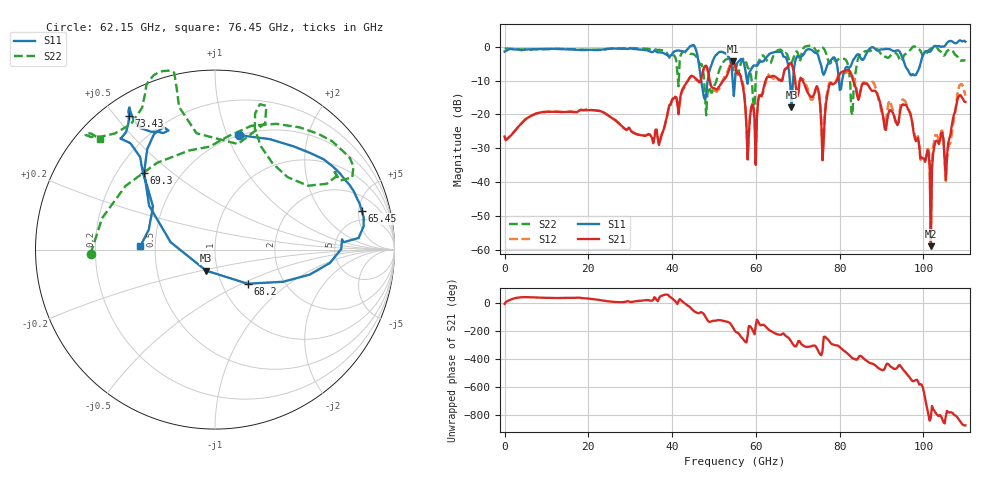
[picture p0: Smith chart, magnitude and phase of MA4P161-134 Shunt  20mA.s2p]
!Keysight Technologies,N5247B,US61255204,A.15.70.20
!Date: Friday, October 21, 2022 14:14:39
!Correction: S11(C  4-Port  )
!S31(C  4-Port  )
!S13(C  4-Port  )
!S33(C  4-Port  )
!S2P File: Measurements: S11, S31, S13, S33:
# Hz S  dB  R 50
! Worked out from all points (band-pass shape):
!   401 points, 10 MHz to 110 GHz, reference 50 ohm
!   highest |S21| = -4.28 dB at 54.46 GHz (marker M1); lowest = -59.0 dB at 101.8 GHz (marker M2)
!   |S21| within 3 dB of the highest: 53.46 GHz to 55.45 GHz (1.988 GHz wide, 3.65 % of centre); 66.75 GHz to 69.02 GHz (2.271 GHz wide, 3.35 % of centre)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
!   lowest |S11| = -17.9 dB at 68.48 GHz (marker M3), VSWR 1.29, Z = 44.1 - j10.5 ohm
!   |S11| at or under -10 dB: 46.93 GHz to 48.49 GHz (1.556 GHz wide, 3.26 % of centre); 54.45 GHz to 55.01 GHz (555.8 MHz wide, 1.02 % of centre); 68.1 GHz to 68.87 GHz (769.8 MHz wide, 1.12 % of centre)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
!   |S22| runs from -20.3 to 0.3 dB; largest |S21 - S12| = 0.16
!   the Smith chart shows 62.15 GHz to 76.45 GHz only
!   S11 on the Smith chart (normalised r, x): 62.15 GHz: 0.50, +1.10; 65.45 GHz: 3.57, +5.42; 68.2 GHz: 1.32, -0.54; 69.3 GHz: 0.31, +0.40; 73.43 GHz: 0.08, +0.54; 76.45 GHz: 0.41, +0.02
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1e7  -1.42 -179.6  -26.54 -8.5  -26.49 -8.4  -0.54 -179.6
1.843332e10  -0.96 130.6  -18.68 32.7  -18.69 32.5  -0.81 140.5
3.685665e10  -1.62 126.2  -29.01 30.6  -28.88 30.6  -0.87 133.7
4.565585e10  -0.71 52.1  -9.40 -67.8  -9.77 -66.4  -2.72 27.1
5.445505e10  -10.08 98.1  -4.28 -174.0  -4.34 -173.9  -5.95 127.6
5.5005e10  -10.01 -177.2  -5.31 158.8  -5.51 158.3  -8.29 148.0
5.802972e10  -10.93 159.8  -33.35 127.2  -33.13 126.0  -6.11 167.5
6.077948e10  -4.68 149.5  -14.31 -149.6  -13.94 -150.7  -4.16 -121.7
6.215435e10  -3.72 78.1  -10.56 -164.9  -11.26 -159.4  -3.17 -178.0
6.545405e10  -1.45 14.8  -9.68 132.1  -9.70 154.0  -0.93 38.1
6.82038e10  -11.59 -46.2  -4.80 93.2  -4.96 90.3  -4.86 45.0
6.847878e10  -17.91 -113.0  -4.98 79.9  -5.18 77.6  -4.76 56.3
6.93037e10  -4.68 132.6  -9.56 48.2  -9.29 47.5  -2.04 73.6
7.342832e10  -1.04 122.7  -14.86 51.8  -15.71 49.9  0.11 111.1
7.645305e10  -7.60 177.5  -20.50 118.3  -19.50 130.5  -1.01 136.1
8.085265e10  -8.24 -75.5  -7.23 21.1  -7.65 21.4  -3.50 -144.2
8.305245e10  -4.38 -45.6  -9.31 -36.6  -8.76 -20.5  -20.18 13.9
8.607718e10  -2.80 6.4  -10.87 -47.1  -10.72 -46.0  -1.28 -14.7
9.185165e10  -0.68 71.6  -18.82 -85.9  -15.85 -82.9  -3.01 67.2
9.762612e10  -8.21 177.6  -25.25 158.9  -24.76 156.9  0.14 166.0
1.017508e11  -1.23 -88.1  -58.97 -99.9  -55.90 -83.6  -0.52 -124.5
1.1e11  1.51 8.1  -16.31 -156.0  -14.40 -161.1  -4.05 16.4
